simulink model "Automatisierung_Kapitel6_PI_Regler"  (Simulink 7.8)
settings: Solver=ode45  StartTime=0.0  StopTime=3  MaxStep=0.2  RelTol=1e-3
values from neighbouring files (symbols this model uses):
  Ad = RzSS.a    [AT_Kapitel6_Diskreter_PI_Reglerentwurf.m]
  Bd = RzSS.b    [AT_Kapitel6_Diskreter_PI_Reglerentwurf.m]
  Cd = RzSS.c    [AT_Kapitel6_Diskreter_PI_Reglerentwurf.m]
  Dd = RzSS.d    [AT_Kapitel6_Diskreter_PI_Reglerentwurf.m]
  Ta = 0.15    [AT_Kapitel6_Diskreter_PI_Reglerentwurf.m]
libraries: cstblocks x1

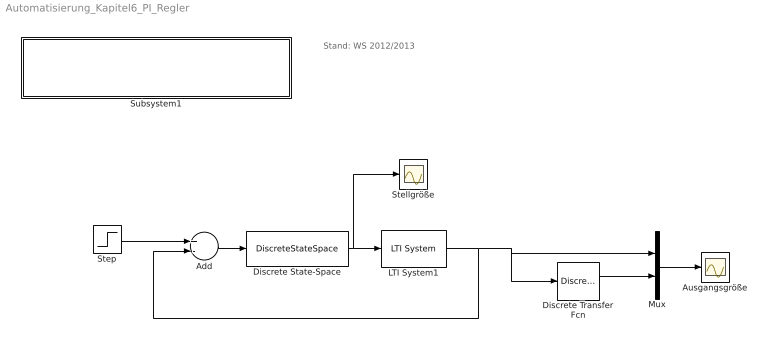
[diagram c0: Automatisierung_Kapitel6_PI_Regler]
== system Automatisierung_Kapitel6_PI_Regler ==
  note: Stand: WS 2012/2013
  Add : Sum  Inputs=+-
  Ausgangsgröße : Scope
  Discrete Transfer Fcn : DiscreteTransferFcn  Denominator=[1]  SampleTime=Ta
  Discrete State-Space : DiscreteStateSpace  A=Ad  B=Bd  C=Cd  D=Dd  SampleTime=Ta
  LTI System1 : cstblocks/LTI System  sys=Gs  IC=[]
  Mux : Mux  Inputs=2
  Stellgröße : Scope
  Step : Step  Time=0  SampleTime=0
  Subsystem1 : Subsystem  Description=asas
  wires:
  Discrete State-Space/1 -> LTI System1/1, Stellgröße/1
  LTI System1/1 -> Add/2, Discrete Transfer Fcn/1, Mux/1
  Add/1 -> Discrete State-Space/1
  Step/1 -> Add/1
  Discrete Transfer Fcn/1 -> Mux/2
  Mux/1 -> Ausgangsgröße/1

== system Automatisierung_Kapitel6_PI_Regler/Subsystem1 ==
